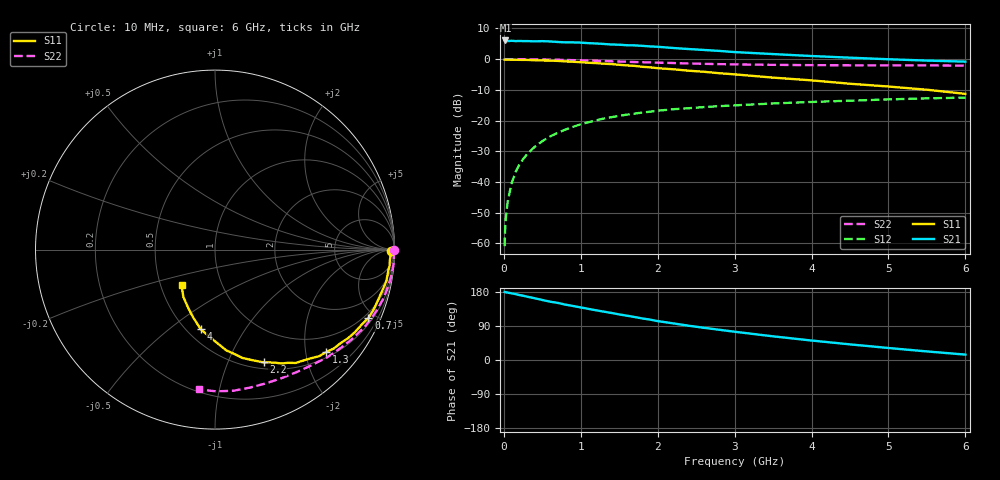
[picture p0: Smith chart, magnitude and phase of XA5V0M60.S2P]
! SIEMENS Discrete & RF Semiconductors
! BFY180
! Si NPN RF Bipolar Junction Transistor in MICRO-X
! VCE = 5 V  IC = 0.6 mA
! Common Emitter S-Parameters:  May  1997
# GHz  S  MA  R  50
!  f  S11  S21  S12  S22
! GHz  MAG  ANG  MAG  ANG  MAG  ANG  MAG  ANG
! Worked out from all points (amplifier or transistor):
!   36 points, 10 MHz to 6 GHz, reference 50 ohm
!   highest |S21| = 6.1 dB at 20 MHz (marker M1)
!   |S21| within 3 dB of that: start of sweep to 2.539 GHz
!   unconditionally stable (mu >= 1): 5.456 GHz to end of sweep
!   at 250 MHz: K = 0.06, MSG = 19.2 dB, |S12| = -32.6 dB
!   at 1.4 GHz: K = 0.41, MSG = 11.8 dB, |S12| = -18.9 dB
!   at 6 GHz: K = 1.02, MAG = 5.0 dB, |S12| = -12.5 dB
!   S11 on the Smith chart (normalised r, x): 10 MHz: open; 700 MHz: 0.75, -4.59; 1.3 GHz: 0.62, -2.42; 2.2 GHz: 0.57, -1.36; 4 GHz: 0.58, -0.65; 6 GHz: 0.64, -0.27
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0.01  0.9811 -0.3  1.988 179.5  0.0009 88.7  0.9983 -0.2
0.02  0.9782 -0.7  2.013 178.9  0.0022 96.3  0.9987 -0.4
0.05  0.9792 -1.7  1.964 177.9  0.0048 86.6  0.9985 -1.2
0.1  0.9763 -3.4  1.99 175.9  0.0094 90.1  0.9963 -2.4
0.15  0.9764 -5.4  1.967 173.9  0.0143 87.2  0.9988 -3.5
0.2  0.9728 -6.9  1.971 171.5  0.0189 84.6  0.9975 -4.6
0.3  0.971 -10.4  1.966 167.2  0.0281 82.8  0.9942 -7.0
0.4  0.9593 -13.9  1.948 163.0  0.0372 80.0  0.9922 -9.3
0.6  0.9458 -20.5  1.941 153.9  0.0549 74.3  0.9822 -13.8
0.7  0.9355 -24.0  1.902 150.7  0.0631 71.8  0.977 -16.1
0.9  0.9053 -30.5  1.874 142.5  0.0791 66.4  0.9624 -20.4
1.1  0.8725 -36.7  1.819 134.9  0.0938 61.9  0.947 -24.6
1.3  0.8419 -42.8  1.765 127.6  0.1078 57.4  0.9308 -28.7
1.8  0.7497 -57.3  1.644 109.7  0.1349 48.0  0.8899 -37.9
2.2  0.6839 -66.7  1.518 96.7  0.1527 41.0  0.864 -44.6
2.4  0.6478 -71.7  1.46 90.5  0.1586 38.2  0.8484 -47.6
2.8  0.5892 -79.8  1.36 79.8  0.1715 33.0  0.8286 -53.3
3.5  0.4996 -91.6  1.208 62.4  0.1897 25.3  0.8069 -62.5
4  0.4511 -100.1  1.123 51.4  0.2006 20.4  0.7975 -69.1
4.5  0.3972 -107.8  1.055 41.2  0.2106 16.0  0.7932 -75.7
5.5  0.3175 -123.7  0.946 22.6  0.2295 7.2  0.7897 -89.6
6  0.2716 -133.4  0.91 14.2  0.2365 2.7  0.7839 -96.5
